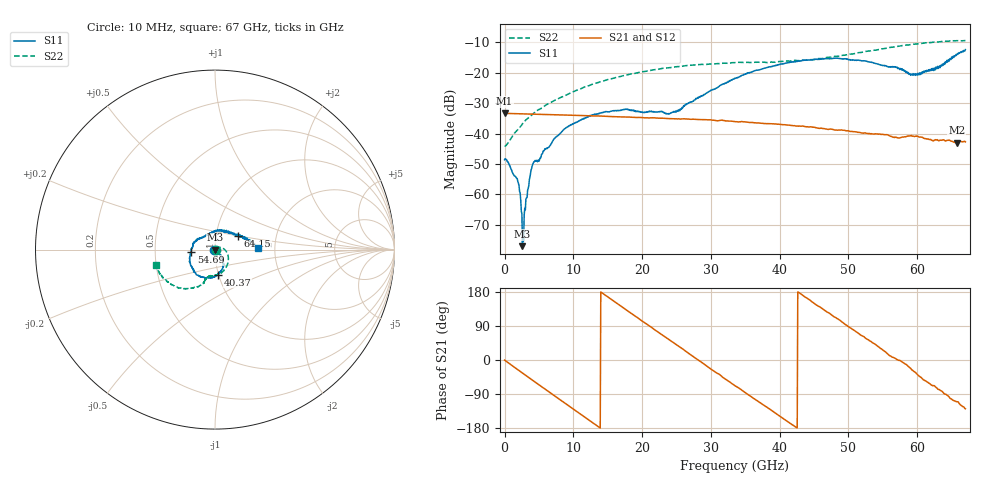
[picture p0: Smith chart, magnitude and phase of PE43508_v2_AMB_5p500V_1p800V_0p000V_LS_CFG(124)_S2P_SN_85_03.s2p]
!Keysight Technologies,N5227A,US51270237,A.10.43.00
!Date: Wednesday, August 22, 2018 17:19:39
!Correction: S11(Full 2 Port(1,3))
!S31(Full 2 Port(1,3))
!S13(Full 2 Port(1,3))
!S33(Full 2 Port(1,3))
!S2P File: Measurements: S11, S31, S13, S33:
# Hz S  dB  R 50
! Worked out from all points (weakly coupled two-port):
!   801 points, 10 MHz to 67 GHz, reference 50 ohm
!   highest |S21| = -33.31 dB at 10 MHz (marker M1); lowest = -43.0 dB at 65.74 GHz (marker M2)
!   lowest |S11| = -77.0 dB at 2.606 GHz (marker M3), VSWR 1.00, Z = 50 - j0.00466 ohm
!   |S11| at or under -10 dB: start of sweep to end of sweep
!   |S22| runs from -44.1 to -9.4 dB; largest |S21 - S12| = 0.00013
!   S11 on the Smith chart (normalised r, x): 10 MHz: 0.99, -0.00; 40.37 GHz: 0.99, -0.28; 54.69 GHz: 0.77, -0.02; 64.15 GHz: 1.27, +0.19; 67 GHz: 1.63, +0.03
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1e7  -48.57 -175.0  -33.31 -0.3  -33.32 -0.2  -44.06 -1.2
1.852225e9  -54.86 160.5  -33.45 -24.7  -33.45 -24.7  -38.87 34.7
2.187175e9  -59.02 174.2  -33.47 -29.0  -33.47 -29.1  -38.04 34.6
2.605862e9  -76.99 -160.8  -33.50 -34.5  -33.50 -34.5  -36.78 34.4
2.940812e9  -64.52 -18.4  -33.52 -38.9  -33.52 -38.9  -35.87 34.6
3.192025e9  -61.13 -18.2  -33.54 -42.1  -33.54 -42.1  -35.34 34.6
3.69445e9  -54.29 -38.4  -33.57 -48.6  -33.57 -48.6  -34.39 32.7
4.280612e9  -49.22 -27.9  -33.60 -56.1  -33.61 -56.2  -33.21 31.0
8.634962e9  -38.64 -60.9  -33.88 -112.0  -33.87 -112.0  -27.68 12.6
1.123082e10  -35.26 -68.7  -34.05 -145.2  -34.06 -145.2  -25.08 -2.5
1.74274e10  -32.08 -87.8  -34.50 135.9  -34.50 135.9  -20.87 -34.2
2.236791e10  -32.79 -82.1  -34.92 73.0  -34.92 73.0  -18.83 -56.6
2.513125e10  -32.34 -64.1  -35.16 38.5  -35.16 38.4  -17.94 -67.2
3.3505e10  -21.87 -55.9  -36.04 -68.0  -36.04 -68.1  -16.65 -92.8
4.037148e10  -17.05 -83.6  -37.04 -152.7  -37.02 -152.7  -16.24 -103.0
4.472582e10  -15.75 -106.7  -37.83 153.3  -37.85 153.3  -15.68 -105.8
5.469059e10  -17.49 -174.8  -40.24 30.2  -40.21 29.9  -12.20 -119.5
5.586291e10  -18.17 171.5  -40.59 13.2  -40.57 12.7  -11.74 -122.9
5.979858e10  -20.34 113.3  -40.80 -33.9  -40.79 -34.1  -10.57 -135.2
6.415292e10  -16.66 30.2  -42.40 -90.4  -42.41 -90.6  -9.63 -152.4
6.574394e10  -14.11 13.6  -42.96 -110.1  -43.04 -110.6  -9.46 -159.0
6.7e10  -12.37 1.8  -42.71 -128.8  -42.78 -129.1  -9.38 -165.3
